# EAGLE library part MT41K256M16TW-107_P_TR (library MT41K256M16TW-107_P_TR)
DRAM DDR3 4G 256MX16 FBGA Source: Datasheet
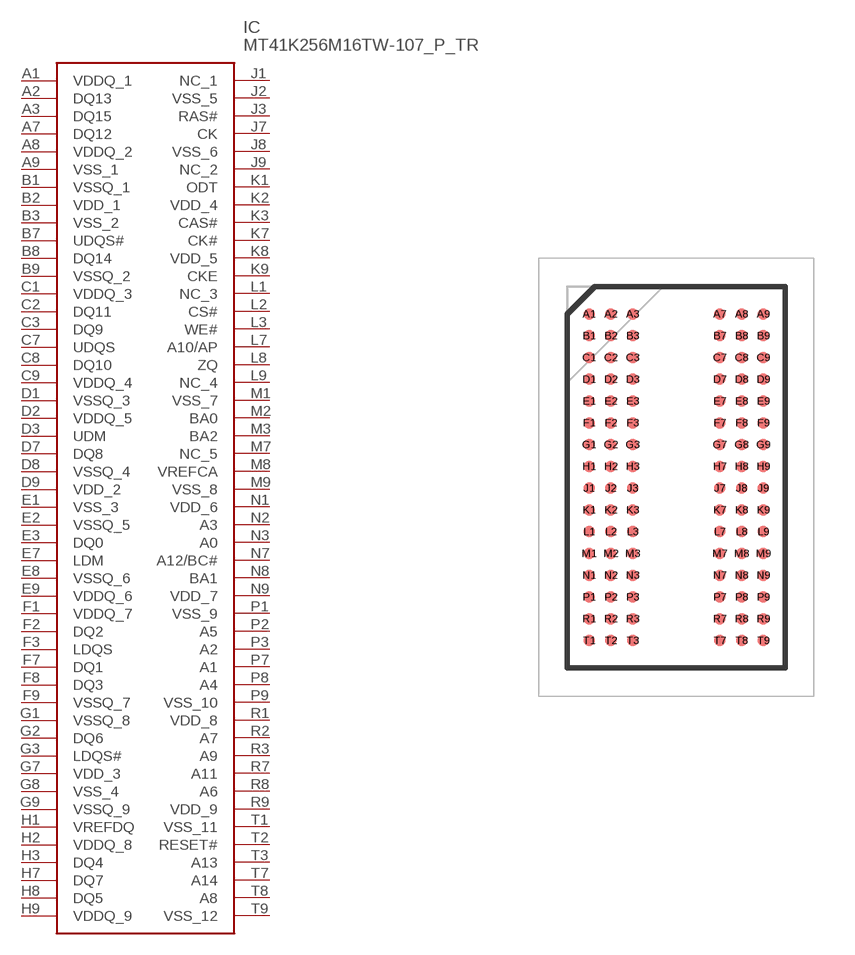
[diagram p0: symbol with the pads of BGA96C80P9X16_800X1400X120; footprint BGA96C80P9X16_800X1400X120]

Designator prefix IC

## MT41K256M16TW-107_P_TR (Description: DRAM DDR3 4G 256MX16 FBGA; Height: 1.2mm; Manufacturer_Name: Micron; Manufacturer_Part_Number: MT41K256M16TW-107:P TR; Mouser_Part_Number: 340-265846-REEL; Mouser_Price-Stock: https://www.mouser.co.uk/ProductDetail/Micron/MT41K256M16TW-107P-TR?qs=j%252B1pi9TdxUafSkKsJ9J8mQ%3D%3D)  [BGA96C80P9X16_800X1400X120]
A1  VDDQ_1
A2  DQ13
A3  DQ15
A7  DQ12
A8  VDDQ_2
A9  VSS_1
B1  VSSQ_1
B2  VDD_1
B3  VSS_2
B7  UDQS#
B8  DQ14
B9  VSSQ_2
C1  VDDQ_3
C2  DQ11
C3  DQ9
C7  UDQS
C8  DQ10
C9  VDDQ_4
D1  VSSQ_3
D2  VDDQ_5
D3  UDM
D7  DQ8
D8  VSSQ_4
D9  VDD_2
E1  VSS_3
E2  VSSQ_5
E3  DQ0
E7  LDM
E8  VSSQ_6
E9  VDDQ_6
F1  VDDQ_7
F2  DQ2
F3  LDQS
F7  DQ1
F8  DQ3
F9  VSSQ_7
G1  VSSQ_8
G2  DQ6
G3  LDQS#
G7  VDD_3
G8  VSS_4
G9  VSSQ_9
H1  VREFDQ
H2  VDDQ_8
H3  DQ4
H7  DQ7
H8  DQ5
H9  VDDQ_9
J1  NC_1
J2  VSS_5
J3  RAS#
J7  CK
J8  VSS_6
J9  NC_2
K1  ODT
K2  VDD_4
K3  CAS#
K7  CK#
K8  VDD_5
K9  CKE
L1  NC_3
L2  CS#
L3  WE#
L7  A10/AP
L8  ZQ
L9  NC_4
M1  VSS_7
M2  BA0
M3  BA2
M7  NC_5
M8  VREFCA
M9  VSS_8
N1  VDD_6
N2  A3
N3  A0
N7  A12/BC#
N8  BA1
N9  VDD_7
P1  VSS_9
P2  A5
P3  A2
P7  A1
P8  A4
P9  VSS_10
R1  VDD_8
R2  A7
R3  A9
R7  A11
R8  A6
R9  VDD_9
T1  VSS_11
T2  RESET#
T3  A13
T7  A14
T8  A8
T9  VSS_12

## Footprint BGA96C80P9X16_800X1400X120 (pad centres in mm)
96-Ball FBGA &ndash; x16 (TW)
smd 0.426 x 0.426: A1 -3.2,6; A2 -2.4,6; A3 -1.6,6; A7 1.6,6; A8 2.4,6; A9 3.2,6; B1 -3.2,5.2; B2 -2.4,5.2; B3 -1.6,5.2; B7 1.6,5.2; B8 2.4,5.2; B9 3.2,5.2; C1 -3.2,4.4; C2 -2.4,4.4; C3 -1.6,4.4; C7 1.6,4.4; C8 2.4,4.4; C9 3.2,4.4; D1 -3.2,3.6; D2 -2.4,3.6; D3 -1.6,3.6; D7 1.6,3.6; D8 2.4,3.6; D9 3.2,3.6; E1 -3.2,2.8; E2 -2.4,2.8; E3 -1.6,2.8; E7 1.6,2.8; E8 2.4,2.8; E9 3.2,2.8; F1 -3.2,2; F2 -2.4,2; F3 -1.6,2; F7 1.6,2; F8 2.4,2; F9 3.2,2; G1 -3.2,1.2; G2 -2.4,1.2; G3 -1.6,1.2; G7 1.6,1.2; G8 2.4,1.2; G9 3.2,1.2; H1 -3.2,0.4; H2 -2.4,0.4; H3 -1.6,0.4; H7 1.6,0.4; H8 2.4,0.4; H9 3.2,0.4; J1 -3.2,-0.4; J2 -2.4,-0.4; J3 -1.6,-0.4; J7 1.6,-0.4; J8 2.4,-0.4; J9 3.2,-0.4; K1 -3.2,-1.2; K2 -2.4,-1.2; K3 -1.6,-1.2; K7 1.6,-1.2; K8 2.4,-1.2; K9 3.2,-1.2; L1 -3.2,-2; L2 -2.4,-2; L3 -1.6,-2; L7 1.6,-2; L8 2.4,-2; L9 3.2,-2; M1 -3.2,-2.8; M2 -2.4,-2.8; M3 -1.6,-2.8; M7 1.6,-2.8; M8 2.4,-2.8; M9 3.2,-2.8; N1 -3.2,-3.6; N2 -2.4,-3.6; N3 -1.6,-3.6; N7 1.6,-3.6; N8 2.4,-3.6; N9 3.2,-3.6; P1 -3.2,-4.4; P2 -2.4,-4.4; P3 -1.6,-4.4; P7 1.6,-4.4; P8 2.4,-4.4; P9 3.2,-4.4; R1 -3.2,-5.2; R2 -2.4,-5.2; R3 -1.6,-5.2; R7 1.6,-5.2; R8 2.4,-5.2; R9 3.2,-5.2; T1 -3.2,-6; T2 -2.4,-6; T3 -1.6,-6; T7 1.6,-6; T8 2.4,-6; T9 3.2,-6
